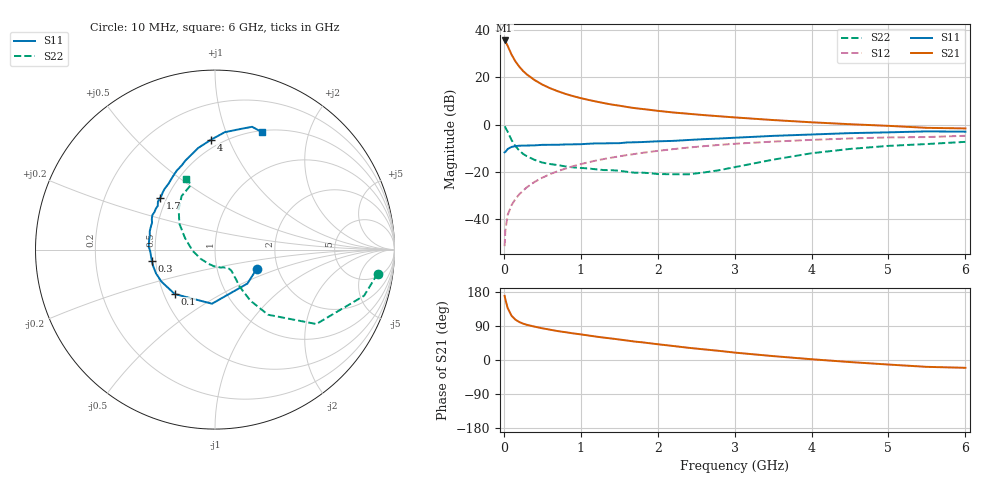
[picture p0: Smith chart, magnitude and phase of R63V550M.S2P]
! SIEMENS Small Signal Semiconductors
! BFR193
! Si NPN RF Bipolar Junction Transistor in SOT23
! VCE = 3.5 V  IC = 50 mA
! Common Emitter S-Parameters:  May  1996
# GHz  S  MA  R  50
!  f  S11  S21  S12  S22
! GHz  MAG  ANG  MAG  ANG  MAG  ANG  MAG  ANG
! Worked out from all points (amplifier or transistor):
!   36 points, 10 MHz to 6 GHz, reference 50 ohm
!   highest |S21| = 35.7 dB at 10 MHz (marker M1)
!   |S21| within 3 dB of that: start of sweep to 59.25 MHz
!   unconditionally stable (mu >= 1): 377.2 MHz to 1.913 GHz
!   at 250 MHz: K = 0.96, MSG = 25.4 dB, |S12| = -28.1 dB
!   at 1.4 GHz: K = 1.02, MAG = 10.4 dB, |S12| = -14.1 dB
!   at 6 GHz: K = 0.95, MSG = 1.6 dB, |S12| = -4.8 dB
!   S11 on the Smith chart (normalised r, x): 10 MHz: 1.56, -0.36; 100 MHz: 0.57, -0.32; 300 MHz: 0.48, -0.07; 1.7 GHz: 0.46, +0.32; 4 GHz: 0.44, +0.87; 6 GHz: 0.52, +1.35
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0.01  0.256 -24.6  61.14 169.4  0.0026 85.2  0.9158 -8.4
0.02  0.2617 -46.3  58.38 159.7  0.0056 77.7  0.8695 -17.2
0.05  0.302 -93.2  46.8 137.1  0.012 72.1  0.7005 -36.3
0.1  0.3342 -132.2  30.7 116.9  0.0193 68.0  0.4684 -50.8
0.15  0.3478 -149.2  22.01 106.5  0.0261 70.3  0.3479 -55.2
0.2  0.3544 -158.2  17.01 100.3  0.0329 72.5  0.2801 -56.0
0.25  0.3563 -164.7  13.74 96.0  0.0392 73.6  0.2375 -56.2
0.3  0.3578 -170.2  11.56 92.8  0.0465 74.0  0.2119 -55.1
0.4  0.3603 -177.8  8.801 88.0  0.0604 74.7  0.1772 -53.7
0.5  0.3699 177.3  7.061 83.7  0.0742 74.3  0.1554 -52.5
0.6  0.3705 172.6  5.921 80.0  0.0881 73.8  0.1448 -52.2
0.7  0.3714 167.9  5.11 76.3  0.1018 72.9  0.1374 -53.1
0.8  0.3774 164.4  4.481 73.4  0.1157 71.5  0.1287 -54.4
1.1  0.3904 154.4  3.334 64.7  0.1576 67.9  0.1164 -60.6
1.4  0.4009 145.2  2.659 56.7  0.1977 63.7  0.107 -69.3
1.7  0.4195 136.8  2.233 48.7  0.2366 59.3  0.0946 -82.3
2.2  0.449 125.2  1.804 37.0  0.2997 51.6  0.0878 -115.2
3.5  0.5738 99.4  1.245 10.3  0.4336 31.1  0.1792 158.9
4  0.6137 91.9  1.115 2.0  0.4718 24.0  0.2452 144.0
4.5  0.656 85.3  1.015 -5.4  0.506 16.9  0.3032 131.9
5.5  0.7148 73.2  0.85 -18.1  0.5418 3.1  0.385 110.2
6  0.7046 68.0  0.826 -20.6  0.5765 -0.8  0.4281 112.3
